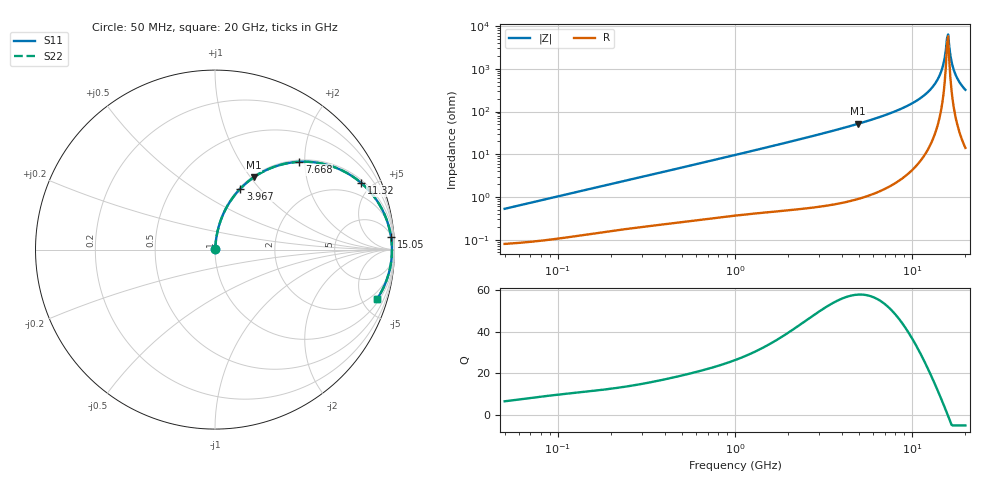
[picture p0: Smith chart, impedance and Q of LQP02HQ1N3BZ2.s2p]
!Murata Part Number: LQP02HQ1N3BZ2
!These Parameters are Measured in Series Mode Connection
!  o--[Z]--o
!Port1  Port2
!  o-------o
!Freq. Start=50[MHz] Stop=20[GHz], 401[Steps]
# Hz S RI R 50
!Freq.(Hz) S11(Real) S11(Imag) S21(Real) S21(Imag) S12(Real) S12(Imag) S22(Real) S22(Imag)
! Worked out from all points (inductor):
!   401 points, 50 MHz to 20 GHz, reference 50 ohm
!   read as one part in series: L = 1.65 nH near 51.52 MHz
!   highest Q = 57.7 at 4.967 GHz (marker M1), where L = 1.66 nH
!   self-resonance near 15.74 GHz
!   S11 on the Smith chart (normalised r, x): 50 MHz: 1.00, +0.01; 3.967 GHz: 1.01, +0.80; 7.668 GHz: 1.04, +1.88; 11.32 GHz: 1.15, +4.31; 15.05 GHz: 6, +26; 20 GHz: 1.28, -6.44
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5e7  0.00082 0.0052  0.9992 -0.0052  0.9992 -0.0052  0.00082 0.0052
1.364002e8  0.00145 0.0138  0.9985 -0.0138  0.9985 -0.0138  0.00145 0.0138
3.721004e8  0.00352 0.0363  0.9965 -0.0363  0.9965 -0.0363  0.00352 0.0363
1e9  0.0126 0.0943  0.9874 -0.0943  0.9874 -0.0943  0.0126 0.0943
2.728004e9  0.0701 0.245  0.9299 -0.245  0.9299 -0.245  0.0701 0.245
3.967106e9  0.1413 0.3395  0.8587 -0.3395  0.8587 -0.3395  0.1413 0.3395
4.966507e9  0.2154 0.4025  0.7846 -0.4025  0.7846 -0.4025  0.2154 0.4025
7.442007e9  0.4463 0.4874  0.5537 -0.4874  0.5537 -0.4874  0.4463 0.4874
7.668323e9  0.4694 0.4892  0.5306 -0.4892  0.5306 -0.4892  0.4694 0.4892
9.457416e9  0.6506 0.4645  0.3494 -0.4645  0.3494 -0.4645  0.6506 0.4645
1.131968e10  0.8145 0.3714  0.1855 -0.3714  0.1855 -0.3714  0.8145 0.3714
1.354865e10  0.9428 0.1997  0.0572 -0.1997  0.0572 -0.1997  0.9428 0.1997
1.438523e10  0.9685 0.128  0.0315 -0.128  0.0315 -0.128  0.9685 0.128
1.504638e10  0.9805 0.0713  0.0195 -0.0713  0.0195 -0.0713  0.9805 0.0713
1.550395e10  0.9847 0.0327  0.0153 -0.0327  0.0153 -0.0327  0.9847 0.0327
1.573793e10  0.9857 0.0132  0.0143 -0.0132  0.0143 -0.0132  0.9857 0.0132
1.597544e10  0.9859 -0.00623  0.0141 0.00623  0.0141 0.00623  0.9859 -0.00623
1.621653e10  0.9853 -0.0257  0.0147 0.0257  0.0147 0.0257  0.9853 -0.0257
1.696185e10  0.979 -0.0837  0.021 0.0837  0.021 0.0837  0.979 -0.0837
1.747767e10  0.971 -0.1215  0.029 0.1215  0.029 0.1215  0.971 -0.1215
1.855685e10  0.9467 -0.194  0.0533 0.194  0.0533 0.194  0.9467 -0.194
2e10  0.9023 -0.2759  0.0977 0.2759  0.0977 0.2759  0.9023 -0.2759
